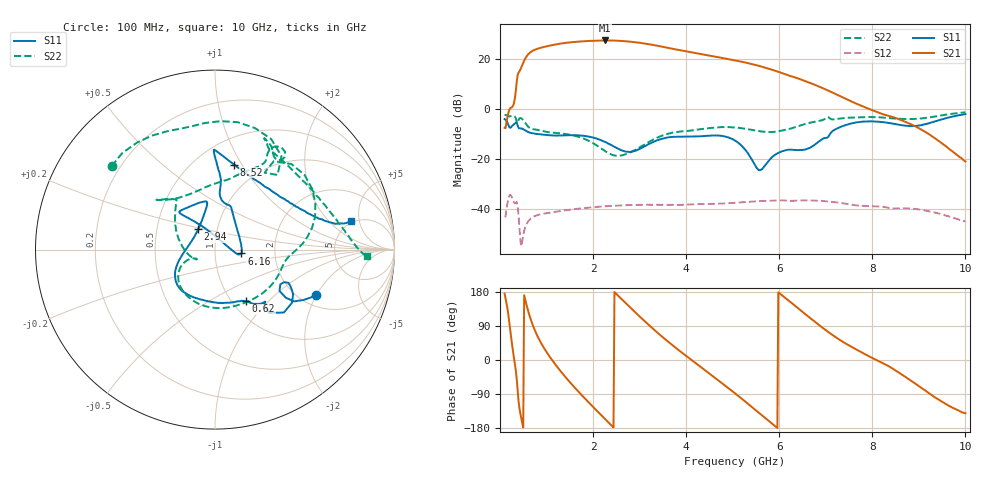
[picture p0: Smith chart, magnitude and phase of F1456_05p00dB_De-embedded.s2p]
! Integrated Device Technology
! Corporate Headquarters
! 6024 Silver Creek Valley Road
! San Jose, CA 95138  USA
! Phone:  1-408-284-8200
! Toll Free:  1-800-223-1366
! Webpage:  http://www.idt.com/
! Timing and RF Division
! 515 Groton Road, Suite 102
! Westford, MA 01886-6024
! Device:  F1456
! Description: 6-bit 0.5 dB Transmit Variable Gain Amplifier
! Frequency:  2100.0 -  2950.00 MHz
! Package:  6x6 mm Thin QFN Plastic Package: 28 pin
! State:  10
! Atten State:  5.0 dB
! Voltage:  +5.00 Volts
! Current:  216.177 mA
! Data:  The device was measured on a the F1455 evaluation board which has
!  individual transmission lines to the RF pins.  Data was collected
!  using a calibrated network analyzer.  The evaluation board was
!  de-embedded using a TRL calibration technique.
!  The reference plane is the edge of the package pin.
!  Pin  1 = CSb
!  Pin  2 = DATA
!  Pin  3 = CLK
!  Pin  4 = RSET
!  Pin  5 = GND
!  Pin  6 = RFIN  = Port 1
!  Pin  7 = GND
!  Pin  8 = NC
!  Pin  9 = NC
!  Pin 10 = NC
!  Pin 11 = NC
!  Pin 12 = NC
!  Pin 13 = NC
!  Pin 14 = /STBY
!  Pin 15 = GND
!  Pin 16 = RFOUT  = Port 2
!  Pin 17 = GND
!  Pin 18 = NC
!  Pin 19 = NC
!  Pin 20 = NC
!  Pin 21 = GND
!  Pin 22 = NC
!  Pin 23 = GND
!  Pin 24 = NC
!  Pin 25 = NC
!  Pin 26 = NC
!  Pin 27 = GND
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# GHz S dB R 50
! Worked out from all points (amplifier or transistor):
!   496 points, 100 MHz to 10 GHz, reference 50 ohm
!   highest |S21| = 27.3 dB at 2.26 GHz (marker M1)
!   |S21| within 3 dB of that: 863.4 MHz to 3.62 GHz (2.757 GHz wide, 123 % of centre)
!   unconditionally stable (mu >= 1): start of sweep to end of sweep
!   at 1.74 GHz: K = 2.09, MAG = 27.5 dB, |S12| = -39.9 dB
!   at 5.06 GHz: K = 3.38, MAG = 20.3 dB, |S12| = -37.7 dB
!   at 10 GHz: K = 118.58, MAG = -11.7 dB, |S12| = -45.2 dB
!   S11 on the Smith chart (normalised r, x): 100 MHz: 2.42, -1.98; 620 MHz: 1.16, -0.75; 2.94 GHz: 0.81, +0.19; 6.16 GHz: 1.34, -0.06; 8.52 GHz: 0.75, +0.92; 10 GHz: 4.77, +3.84
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0.1  -4.19 -24.3  -7.68 175.1  -43.10 43.6  -2.61 141.1
0.34  -5.66 -34.8  6.95 -26.7  -37.75 -143.3  -3.89 54.6
0.42  -7.90 -45.9  14.97 -128.3  -48.00 133.3  -3.89 48.2
0.52  -8.46 -53.2  19.20 171.0  -48.98 -161.1  -5.13 12.6
0.62  -9.47 -58.8  22.00 123.5  -44.84 168.2  -7.49 -3.9
0.8  -10.14 -70.1  23.93 64.7  -42.66 120.6  -8.49 -26.9
1.14  -10.77 -99.0  25.50 -3.5  -41.51 70.2  -9.63 -78.0
1.48  -10.66 -121.5  26.48 -55.4  -40.50 40.3  -10.37 -119.4
1.76  -10.80 -136.5  26.92 -93.2  -39.90 20.8  -11.73 -142.3
2.26  -13.36 -161.7  27.29 -156.1  -39.10 -9.0  -17.01 -159.1
2.58  -16.41 173.3  27.13 164.8  -38.78 -26.6  -18.84 -151.7
2.94  -16.66 129.8  26.50 121.8  -38.53 -45.6  -16.20 -172.2
3.4  -12.56 102.0  25.11 70.4  -38.52 -68.4  -11.48 146.0
4.08  -11.21 111.0  22.61 3.5  -38.38 -96.8  -8.83 129.1
4.58  -10.75 131.7  20.96 -43.4  -38.16 -117.9  -7.64 137.8
5.06  -12.90 129.9  19.29 -88.9  -37.67 -138.0  -7.56 138.7
5.6  -24.52 43.1  16.94 -143.0  -37.01 -166.0  -9.11 123.8
6.16  -16.57 -8.3  13.56 160.7  -36.84 160.3  -8.35 84.2
6.7  -15.26 46.0  10.02 107.2  -36.78 127.8  -5.50 61.9
8.36  -5.75 83.8  -2.93 -16.9  -39.81 50.6  -3.85 62.6
8.52  -6.28 77.5  -3.90 -29.5  -39.95 47.1  -4.02 58.8
10  -2.20 11.9  -21.16 -140.4  -45.19 -30.8  -1.46 -2.5
